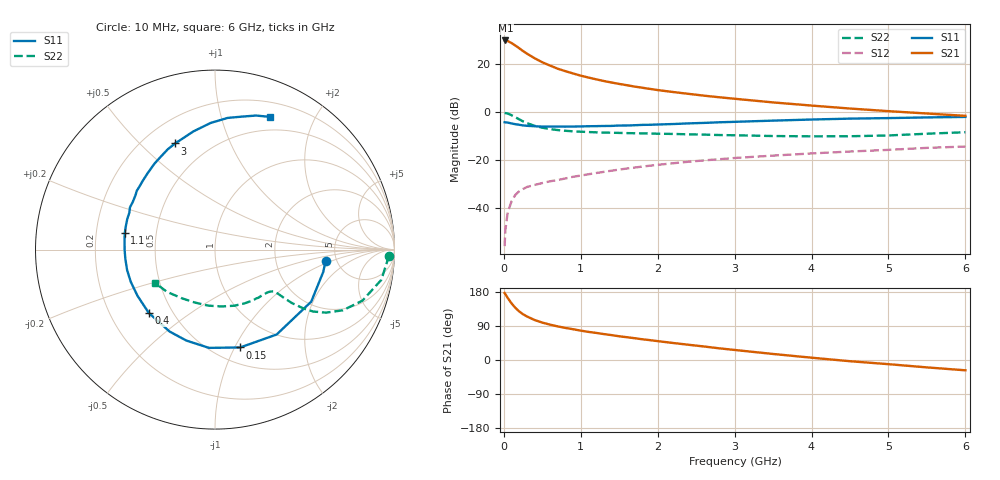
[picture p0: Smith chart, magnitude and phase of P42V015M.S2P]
! SIEMENS Small Signal Semiconductors
! BFP182
! Si NPN RF Bipolar Junction Transistor in SOT143
! VCE = 2 V  IC = 15 mA
! Common Emitter S-Parameters:  March  1996
# GHz  S  MA  R  50
!  f  S11  S21  S12  S22
! GHz  MAG  ANG  MAG  ANG  MAG  ANG  MAG  ANG
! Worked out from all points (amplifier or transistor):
!   36 points, 10 MHz to 6 GHz, reference 50 ohm
!   highest |S21| = 30.0 dB at 20 MHz (marker M1)
!   |S21| within 3 dB of that: start of sweep to 188.7 MHz
!   unconditionally stable (mu >= 1): 827.2 MHz to 5.379 GHz
!   at 250 MHz: K = 0.45, MSG = 28.8 dB, |S12| = -32.0 dB
!   at 1.4 GHz: K = 1.18, MAG = 15.9 dB, |S12| = -24.4 dB
!   at 6 GHz: K = 0.93, MSG = 6.4 dB, |S12| = -14.3 dB
!   S11 on the Smith chart (normalised r, x): 10 MHz: 4.07, -0.84; 150 MHz: 0.66, -1.05; 400 MHz: 0.37, -0.35; 1.1 GHz: 0.33, +0.08; 3 GHz: 0.33, +0.64; 6 GHz: 0.35, +1.44
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0.01  0.6194 -5.9  31.56 176.7  0.0016 85.3  0.9678 -2.0
0.02  0.6157 -11.7  31.61 173.7  0.0035 83.4  0.961 -4.1
0.05  0.6096 -28.4  30.8 163.8  0.0081 80.8  0.9419 -10.3
0.1  0.5846 -54.0  27.9 149.5  0.0138 65.5  0.8693 -19.1
0.15  0.563 -75.6  24.73 137.6  0.0189 59.4  0.7885 -25.4
0.2  0.5485 -93.5  21.73 128.1  0.0224 54.5  0.7111 -29.6
0.25  0.5313 -107.5  18.96 120.7  0.025 51.6  0.6453 -32.3
0.3  0.5219 -119.0  16.8 114.9  0.0275 49.9  0.5935 -33.6
0.4  0.5104 -136.3  13.46 105.5  0.0304 47.9  0.5221 -34.8
0.5  0.5028 -149.1  11.06 98.7  0.0333 46.8  0.476 -35.0
0.6  0.5025 -159.1  9.456 93.3  0.0362 47.2  0.4458 -35.0
0.7  0.5028 -166.9  8.131 88.7  0.0385 48.2  0.4252 -35.0
0.9  0.5035 -179.6  6.468 81.2  0.045 49.5  0.4001 -35.7
1.1  0.5112 169.6  5.315 74.2  0.0508 50.6  0.3866 -37.3
1.5  0.529 153.6  3.906 62.6  0.0636 50.2  0.371 -41.8
1.8  0.5454 143.0  3.253 54.7  0.0734 49.7  0.3629 -46.3
2.2  0.5683 131.1  2.649 44.9  0.0862 47.5  0.3531 -53.5
3  0.6317 110.6  1.916 26.5  0.111 41.5  0.3311 -70.7
3.5  0.6693 100.4  1.607 15.9  0.1245 37.3  0.319 -83.4
4.5  0.7371 84.5  1.197 -3.2  0.1515 29.2  0.3159 -111.4
5.5  0.781 73.0  0.942 -19.5  0.1807 21.1  0.3565 -138.7
6  0.8001 67.6  0.843 -27.2  0.1925 16.0  0.3833 -151.3
